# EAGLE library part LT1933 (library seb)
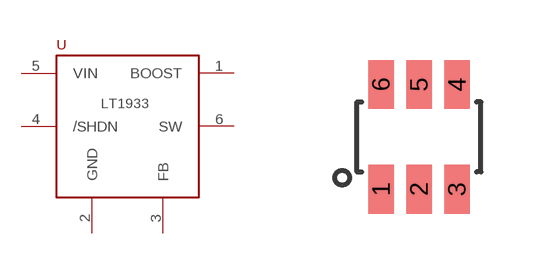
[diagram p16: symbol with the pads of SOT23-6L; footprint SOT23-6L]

Designator prefix -

## LT1933  [SOT23-6L]
1  BOOST
2  GND
3  FB
4  /SHDN
5  VIN
6  SW

## Footprint SOT23-6L (pad centres in mm)
smd 0.63 x 1.22: 1 -0.95,-1.31; 2 0,-1.31; 3 0.95,-1.31; 4 0.95,1.31; 5 0,1.31; 6 -0.95,1.31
